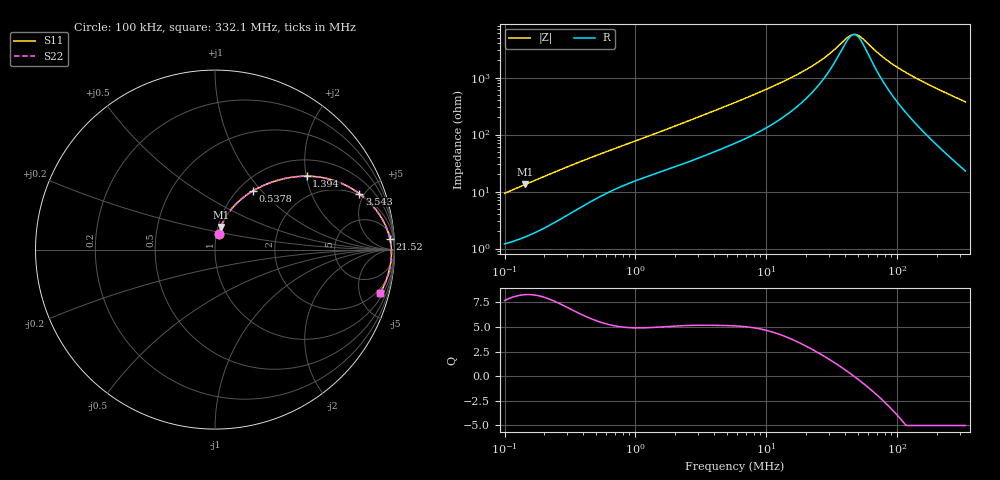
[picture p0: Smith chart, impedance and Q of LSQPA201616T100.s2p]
! LSQPA201616T100  S-PARAMETER MODEL  ( General Type )
! Model Generated by TAIYO YUDEN Corporation (http://www.ty-top.com)
! Version 2.0
! TAIYO YUDEN Control No. 100810NF25SB-FKC
! Copyright(c) 2007 TAIYO YUDEN CO.,LTD. All Rights Reserved.
! Product Description (link to TY-COMPAS)
! https://ds.yuden.co.jp/TYCOMPAS/or/detail?pn=LSQPA201616T100K&u=M
! Products Name : Inductors
! Characteristics :
!  Inductance : 10 uH , SRF(min) : 32 MHz , DC Resistance(max) : 1.066 Ohm
!  Rated Current : Saturation :380 mA , Temp Rise : 350 mA (40 degC)
!  Case Size : 2.0 x 1.6 / 0.079 x 0.063 [mm/inch] , Thickness : 1.6 / 0.063 [mm/inch]
!  (Conditions: Temperature = 25 degC , DC Bias Current/Voltage = 0A / 0V)
! External Node Assignments :
!  1  o---GGG---o  2
! GND o---------o GND
! Frequency Range : 0.1MHz  -  332.076389MHz  [ 402 STEP ]
# MHz S RI R 50
! Freq[MHz].  S11 Real  S11 Imag  S21 Real  S21 Imag  S12 Real  S12 Imag  S22 Real  S22 Imag
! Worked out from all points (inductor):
!   401 points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, 100 kHz to 332.1 MHz, reference 50 ohm
!   read as one part in series: L = 14.7 uH near 104.1 kHz
!   highest Q = 8.28 at 144 kHz (marker M1), where L = 14.6 uH
!   self-resonance near 46.7 MHz
!   S11 on the Smith chart (normalised r, x): 100 kHz: 1.02, +0.18; 537.8 kHz: 1.16, +0.90; 1.394 MHz: 1.41, +2.01; 3.543 MHz: 1.89, +4.60; 21.52 MHz: 11, +28; 332.1 MHz: 1.46, -7.50
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0.1  0.0201 0.0895  0.9799 -0.0895  0.9799 -0.0895  0.0201 0.0895
0.144031  0.0322 0.1261  0.9678 -0.1261  0.9678 -0.1261  0.0322 0.1261
0.24397  0.0707 0.1987  0.9293 -0.1987  0.9293 -0.1987  0.0707 0.1987
0.388873  0.1398 0.2759  0.8602 -0.2759  0.8602 -0.2759  0.1398 0.2759
0.537845  0.2114 0.3273  0.7886 -0.3273  0.7886 -0.3273  0.2114 0.3273
0.91104  0.3635 0.3901  0.6365 -0.3901  0.6365 -0.3901  0.3635 0.3901
1.394448  0.5108 0.4091  0.4892 -0.4091  0.4892 -0.4091  0.5108 0.4091
1.512219  0.5401 0.4081  0.4599 -0.4081  0.4599 -0.4081  0.5401 0.4081
2.222663  0.6743 0.3811  0.3257 -0.3811  0.3257 -0.3811  0.6743 0.3811
3.542784  0.8044 0.3116  0.1956 -0.3116  0.1956 -0.3116  0.8044 0.3116
5.762607  0.8922 0.2273  0.1078 -0.2273  0.1078 -0.2273  0.8922 0.2273
12.19926  0.9569 0.1179  0.0431 -0.1179  0.0431 -0.1179  0.9569 0.1179
21.51891  0.9749 0.0597  0.0251 -0.0597  0.0251 -0.0597  0.9749 0.0597
22.4092  0.9756 0.0562  0.0244 -0.0562  0.0244 -0.0562  0.9756 0.0562
29.76252  0.9797 0.0332  0.0203 -0.0332  0.0203 -0.0332  0.9797 0.0332
42.00706  0.9824 0.00769  0.0176 -0.00769  0.0176 -0.00769  0.9824 0.00769
46.48767  0.9828 0.000335  0.0172 -0.000335  0.0172 -0.000335  0.9828 0.000335
53.57466  0.9831 -0.01  0.0169 0.01  0.0169 0.01  0.9831 -0.01
71.15457  0.9827 -0.0318  0.0173 0.0318  0.0173 0.0318  0.9827 -0.0318
87.14324  0.9816 -0.0488  0.0184 0.0488  0.0184 0.0488  0.9816 -0.0488
150.632  0.9727 -0.1063  0.0273 0.1063  0.0273 0.1063  0.9727 -0.1063
332.0764  0.921 -0.2408  0.079 0.2408  0.079 0.2408  0.921 -0.2408
